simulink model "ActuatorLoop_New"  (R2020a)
settings: Solver=FixedStepDiscrete  StartTime=0.0  StopTime=10.0  FixedStep=0.001  RelTol=1e-3  EnableMultiTasking=on
model workspace (MAT data in the model file):
  Kd : Simulink.Parameter (value not decoded)
  Ki : Simulink.Parameter (value not decoded)
  Kp : Simulink.Parameter (value not decoded)
  Ts : Simulink.Parameter (value not decoded)
symbols that are objects in the model workspace (value not decoded): Kd, Ki, Kp, Ts
undefined symbols (not defined in the file or in its folder): DiscIntNeverNeededParam
libraries: simulink x2

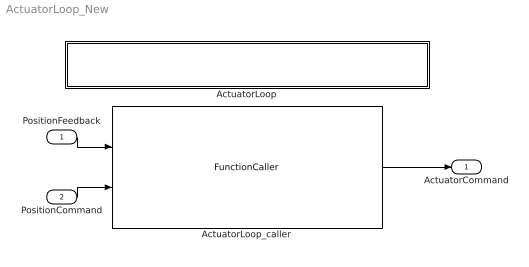
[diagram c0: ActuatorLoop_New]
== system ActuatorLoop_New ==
  PositionFeedback : Inport  OutMin=-32768  OutMax=32767  OutDataTypeStr=int16  PortDimensions=1  SampleTime=0.001
  PositionCommand : Inport  Port=2  OutMin=-0.1  OutMax=0.1  OutDataTypeStr=double  PortDimensions=1  SampleTime=0.001
  ActuatorLoop : Subsystem  TreatAsAtomicUnit=on
  ActuatorLoop_caller : FunctionCaller  FunctionPrototype=ActuatorCommand = ActuatorLoop(PositionFeedback,PositionCommand)  InputArgumentSpecifications=int16(1), double(1)  OutputArgumentSpecifications=int16(1)
  ActuatorCommand : Outport  OutDataTypeStr=int16  PortDimensions=1  SampleTime=0.001  VectorParamsAs1DForOutWhenUnconnected=off
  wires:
  PositionCommand/1 -> ActuatorLoop_caller/2
  PositionFeedback/1 -> ActuatorLoop_caller/1
  ActuatorLoop_caller/1 -> ActuatorCommand/1

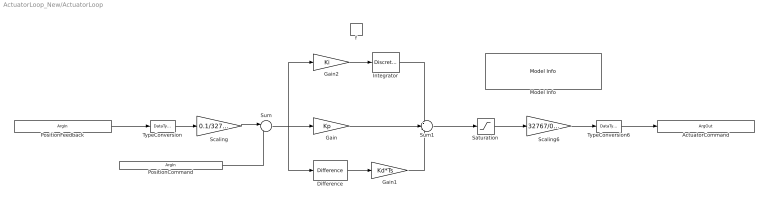
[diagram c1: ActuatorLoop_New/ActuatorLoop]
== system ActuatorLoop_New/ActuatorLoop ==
  f : TriggerPort  TriggerType=function-call  IsSimulinkFunction=on  FunctionName=ActuatorLoop  FunctionVisibility=scoped  VariantControl=Variant  PortDimensions=1
  Difference : simulink/Discrete/Difference  ICPrevInput=0.0  OutMin=[]  OutMax=[]  OutDataType=fixdt(1, 16)  OutScaling=2^-10  DoSatur=off
  Gain : Gain  Gain=Kp
  Gain1 : Gain  Gain=Kd*Ts
  Gain2 : Gain  Gain=Ki
  Integrator : DiscreteIntegrator  SampleTime=-1  LimitOutput=on  UpperSaturationLimit=0.1  LowerSaturationLimit=-0.1  ICPrevOutput=DiscIntNeverNeededParam  ICPrevScaledInput=DiscIntNeverNeededParam
  Model Info : simulink/Model-Wide Utilities/Model Info  Frame=on  DisplayStringWithTags=|  HorizontalTextAlignment=Center  LeftAlignmentValue=0.5
      | Model Name: %<ModelName>
      | Model Version: %<ModelVersion>
      | Last Modified: %<LastModificationDate>
      | 
      | Copyright 2016 The MathWorks, Inc.
  Saturation : Saturate  UpperLimit=0.3  LowerLimit=-0.3
  Scaling : Gain  Gain=0.1/32767
  Scaling6 : Gain  Gain=32767/0.3  SaturateOnIntegerOverflow=on
  Sum : Sum  Inputs=|-+
  Sum1 : Sum  Inputs=++-
  TypeConversion : DataTypeConversion  OutDataTypeStr=double
  TypeConversion6 : DataTypeConversion  OutDataTypeStr=int16
  PositionFeedback : ArgIn  OutMin=-32768  OutMax=32767  OutDataTypeStr=int16  ArgumentName=PositionFeedback
  PositionCommand : ArgIn  Port=2  OutMin=-0.1  OutMax=0.1  ArgumentName=PositionCommand
  ActuatorCommand : ArgOut  OutDataTypeStr=int16  ArgumentName=ActuatorCommand
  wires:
  Gain/1 -> Sum1/2
  PositionCommand/1 -> Sum/2
  Gain2/1 -> Integrator/1
  Scaling6/1 -> TypeConversion6/1
  PositionFeedback/1 -> TypeConversion/1
  Gain1/1 -> Sum1/3
  Sum1/1 -> Saturation/1
  Scaling/1 -> Sum/1
  Sum/1 -> Difference/1, Gain2/1, Gain/1
  Integrator/1 -> Sum1/1
  TypeConversion/1 -> Scaling/1
  TypeConversion6/1 -> ActuatorCommand/1
  Difference/1 -> Gain1/1
  Saturation/1 -> Scaling6/1
